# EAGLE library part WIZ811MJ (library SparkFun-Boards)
WIZnet W%100 Network Module with Mag Jack - WIZ811MJ Mechanical footprint with connectors for WIZ811MJ Breakout board with RJ45 connector. SparkFun Products: WIZ811MJ Breakout
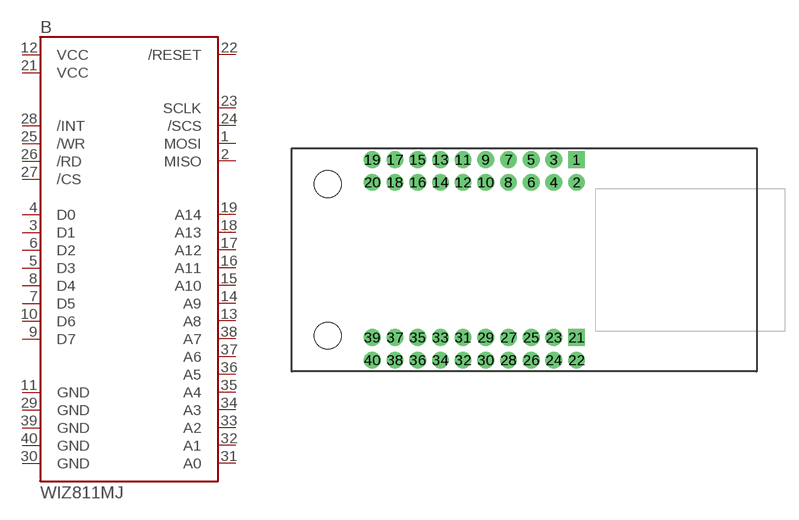
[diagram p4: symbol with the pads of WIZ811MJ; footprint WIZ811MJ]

Designator prefix B

## WIZ811MJ  [WIZ811MJ]
1  MOSI
2  MISO
3  D1
4  D0
5  D3
6  D2
7  D5
8  D4
9  D7
10  D6
11  GND
12  VCC
13  A8
14  A9
15  A10
16  A11
17  A12
18  A13
19  A14
21  VCC
22  /RESET
23  SCLK
24  /SCS
25  /WR
26  /RD
27  /CS
28  /INT
29  GND
30  GND
31  A0
32  A1
33  A2
34  A3
35  A4
36  A5
37  A6
38  A7
39  GND
40  GND

## Footprint WIZ811MJ (pad centres in mm)
WIZnet W5100 Network Module with MagJack - WIZ811MJ Footprint Specifications: Pin count:40 Pin pitch: 0.1" Area:2.05x1.0" Example device(s): WIZNet
drill 1.02 pad 1.88 square: 1 6.35,11.43; 21 6.35,-8.49
drill 1.02 pad 1.88: 2 6.35,8.89; 3 3.81,11.43; 4 3.81,8.89; 5 1.27,11.43; 6 1.27,8.89; 7 -1.27,11.43; 8 -1.27,8.89; 9 -3.81,11.43; 10 -3.81,8.89; 11 -6.35,11.43; 12 -6.35,8.89; 13 -8.89,11.43; 14 -8.89,8.89; 15 -11.43,11.43; 16 -11.43,8.89; 17 -13.97,11.43; 18 -13.97,8.89; 19 -16.51,11.43; 20 -16.51,8.89; 22 6.35,-11.03; 23 3.81,-8.49; 24 3.81,-11.03; 25 1.27,-8.49; 26 1.27,-11.03; 27 -1.27,-8.49; 28 -1.27,-11.03; 29 -3.81,-8.49; 30 -3.81,-11.03; 31 -6.35,-8.49; 32 -6.35,-11.03; 33 -8.89,-8.49; 34 -8.89,-11.03; 35 -11.43,-8.49; 36 -11.43,-11.03; 37 -13.97,-8.49; 38 -13.97,-11.03; 39 -16.51,-8.49; 40 -16.51,-11.03
hole 3 at -21.51,-8.3
hole 3 at -21.51,8.7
